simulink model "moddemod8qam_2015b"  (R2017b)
settings: Solver=VariableStepAuto  StartTime=0.0  StopTime=10.0  RelTol=1e-3
libraries: commdigbbndam3 x2, commrandsrc3 x1, dspsrcs4 x1

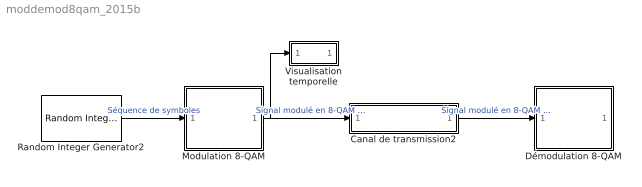
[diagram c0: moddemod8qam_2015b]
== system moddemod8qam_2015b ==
  Canal de transmission2 : Subsystem
  Démodulation 8-QAM : Subsystem
  Modulation 8-QAM : Subsystem
  Random Integer Generator2 : commrandsrc3/Random Integer Generator  SetSize=8  SeedSource=Auto  Seed=0  SampleTime=1  SamplesPerFrame=1  OutputDataType=double  SimulateUsing=Interpreted execution
  Visualisation temporelle : Subsystem
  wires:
  Modulation 8-QAM/1(Out1) -> Canal de transmission2/1(In1), Visualisation temporelle/1(In1)  "Signal modulé en 8-QAM émis"
  Visualisation temporelle/1(Out1) -> ?  "Signal modulé en 8-QAM émis"
  Random Integer Generator2/1 -> Modulation 8-QAM/1(In1)  "Séquence de symboles"
  Canal de transmission2/1(Out1) -> Démodulation 8-QAM/1(In1)  "Signal modulé en 8-QAM reçu"
  Démodulation 8-QAM/1(Out1) -> ?  "Séquence de symboles démodulé"

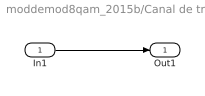
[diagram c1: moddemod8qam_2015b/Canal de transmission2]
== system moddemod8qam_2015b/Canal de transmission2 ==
  In1 : Inport
  Out1 : Outport
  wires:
  In1/1 -> Out1/1

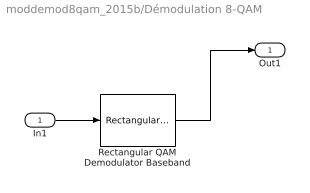
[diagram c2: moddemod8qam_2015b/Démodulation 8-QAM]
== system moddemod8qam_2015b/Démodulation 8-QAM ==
  In1 : Inport
  Rectangular QAM Demodulator Baseband : commdigbbndam3/Rectangular QAM Demodulator Baseband  M=8  OutType=Integer  DecType=Hard decision  VarSource=Dialog  Variance=1  Dec=Binary  Mapping=[0:15]  PowType=Min. distance between symbols  MinDist=2  AvgPow=1  PeakPow=1  Ph=0  outDtype1=Inherit via internal rule  outDtype2=Inherit via internal rule  derotateFactorWordLen=16  derotateFactorDataTypeStr=Inherit: Same word length as input  derotateFactorLastDataTypeStr=Inherit: Same word length as input  denormFactorWordLen=16  denormFactorDataTypeStr=Inherit: Same word length as input  denormFactorLastDataTypeStr=Inherit: Same word length as input  prodOutWordLen=32  prodOutOverflowMode=Wrap  prodOutRoundingMode=Floor  prodOutOvFlMode=off  prodOutOvFlModeLastStrValue=off  sumWordLen=32
  Out1 : Outport
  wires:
  Rectangular QAM Demodulator Baseband/1 -> Out1/1
  In1/1 -> Rectangular QAM Demodulator Baseband/1

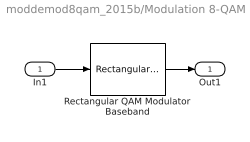
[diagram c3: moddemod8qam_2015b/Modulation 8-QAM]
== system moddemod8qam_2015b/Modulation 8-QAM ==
  In1 : Inport
  Rectangular QAM Modulator Baseband : commdigbbndam3/Rectangular QAM Modulator Baseband  M=8  InType=Integer  Enc=Binary  Mapping=[0:15]  PowType=Min. distance between symbols  MinDist=2  AvgPow=1  PeakPow=1  Ph=0  outDtype=double  outWordLen=16  outUDDataType=sfix(16)  outFracLenMode=Best precision  outFracLen=15  outDataTypeStr=double  outLastDataTypeStr=double
  Out1 : Outport
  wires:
  Rectangular QAM Modulator Baseband/1 -> Out1/1
  In1/1 -> Rectangular QAM Modulator Baseband/1

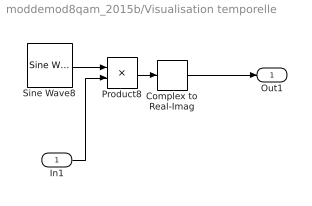
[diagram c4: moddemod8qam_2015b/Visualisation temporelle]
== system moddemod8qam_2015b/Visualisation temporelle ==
  In1 : Inport
  Complex to Real-Imag : ComplexToRealImag  Output=Real
  Product8 : Product
  Sine Wave8 : dspsrcs4/Sine Wave  Amplitude=1  Frequency=1  Phase=0  SampleMode=Discrete  OutComplex=Complex  CompMethod=Trigonometric fcn  TableSize=Speed  SampleTime=1/100  SamplesPerFrame=1  ResetState=Restart at time zero  OutputFrames=off  dataType=double  wordLen=16  udDataType=sfix(16)  fracBitsMode=Best precision  numFracBits=15  OutDataTypeStr=double  LastOutDataTypeStr=double
  Out1 : Outport
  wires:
  Product8/1 -> Complex to Real-Imag/1
  Sine Wave8/1 -> Product8/1
  In1/1 -> Product8/2
  Complex to Real-Imag/1 -> Out1/1
